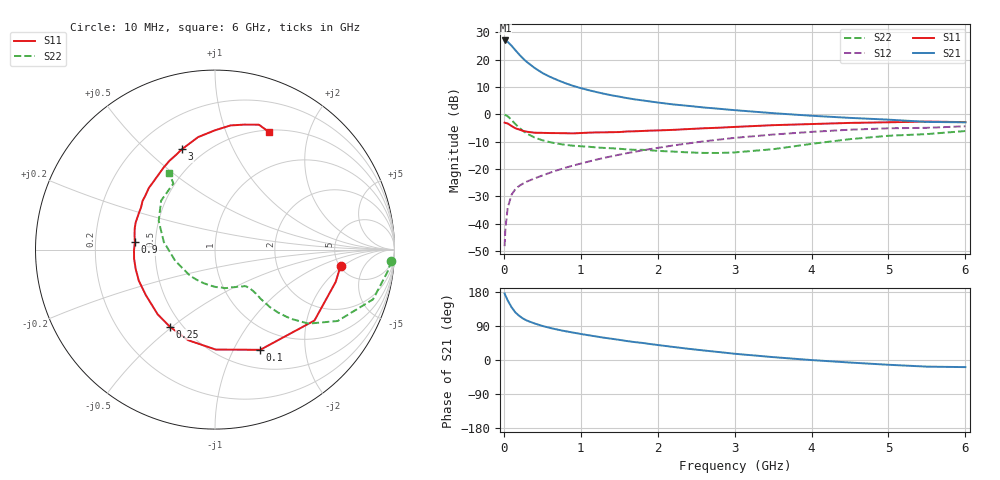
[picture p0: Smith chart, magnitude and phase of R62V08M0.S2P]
! SIEMENS Small Signal Semiconductors
! BFR193
! Si NPN RF Bipolar Junction Transistor in SOT23
! VCE = 2 V  IC = 8 mA
! Common Emitter S-Parameters:  May  1996
# GHz  S  MA  R  50
!  f  S11  S21  S12  S22
! GHz  MAG  ANG  MAG  ANG  MAG  ANG  MAG  ANG
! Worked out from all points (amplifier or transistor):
!   36 points, 10 MHz to 6 GHz, reference 50 ohm
!   highest |S21| = 27.0 dB at 20 MHz (marker M1)
!   |S21| within 3 dB of that: start of sweep to 133 MHz
!   unconditionally stable (mu >= 1): 773.6 MHz to 2.024 GHz
!   at 250 MHz: K = 0.57, MSG = 22.8 dB, |S12| = -25.3 dB
!   at 1.4 GHz: K = 1.05, MAG = 9.8 dB, |S12| = -15.3 dB
!   at 6 GHz: K = 0.96, MSG = 0.7 dB, |S12| = -4.4 dB
!   lowest NFmin = 1.25 dB at 450 MHz
!   S11 on the Smith chart (normalised r, x): 10 MHz: 5.08, -1.86; 100 MHz: 0.72, -1.28; 250 MHz: 0.43, -0.49; 900 MHz: 0.38, +0.04; 3 GHz: 0.38, +0.65; 6 GHz: 0.52, +1.43
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0.01  0.7054 -7.5  22.26 175.5  0.0039 86.8  0.9853 -3.6
0.02  0.6961 -15.0  22.37 170.4  0.008 81.8  0.9695 -7.3
0.05  0.6806 -35.5  21.09 157.4  0.0195 73.9  0.9229 -17.5
0.1  0.6126 -65.7  17.95 139.4  0.0339 63.2  0.7907 -30.2
0.15  0.5569 -89.6  14.85 125.6  0.043 56.4  0.6641 -38.4
0.2  0.5265 -106.5  12.38 116.5  0.0493 53.4  0.5687 -42.5
0.25  0.4978 -120.4  10.45 109.4  0.0543 52.1  0.4981 -44.9
0.3  0.4816 -131.6  9.028 104.0  0.0591 52.6  0.4445 -46.3
0.4  0.4613 -146.8  7.042 96.4  0.0675 53.6  0.3763 -47.1
0.5  0.4586 -157.7  5.708 90.0  0.0762 55.1  0.3361 -47.1
0.6  0.4549 -166.4  4.843 84.7  0.0857 56.6  0.3096 -47.4
0.7  0.4536 -173.7  4.212 80.1  0.0956 58.4  0.2909 -48.1
0.9  0.4484 174.7  3.314 72.3  0.1158 59.9  0.2671 -49.9
1.1  0.4627 165.1  2.768 65.4  0.1369 60.7  0.2559 -53.4
1.3  0.4683 157.0  2.38 58.9  0.1598 60.3  0.2435 -57.5
1.6  0.486 146.2  1.981 50.0  0.1951 59.1  0.2288 -66.2
2.2  0.52 128.1  1.517 34.5  0.2695 54.0  0.2086 -88.6
3  0.5886 108.3  1.192 16.5  0.3717 43.5  0.2014 -133.8
3.5  0.6336 98.6  1.05 7.6  0.427 35.8  0.2306 -164.5
4.5  0.6971 82.9  0.861 -6.7  0.5235 20.5  0.352 153.0
5.5  0.7377 70.6  0.727 -17.5  0.5672 4.6  0.4353 122.2
6  0.7207 65.3  0.714 -18.8  0.6048 -0.1  0.4953 120.9
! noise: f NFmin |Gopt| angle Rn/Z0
0.45  1.25  0.23  133  0.12
0.9  1.3  0.35  156  0.11
1.8  2  0.55  -155  0.13
